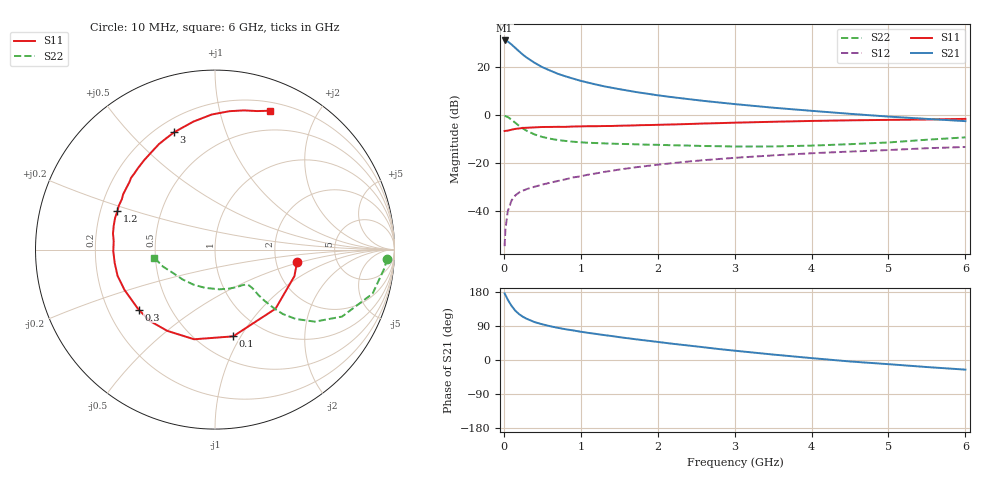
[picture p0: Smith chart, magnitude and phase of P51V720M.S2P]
! SIEMENS Small Signal Semiconductors
! BFP183
! Si NPN RF Bipolar Junction Transistor in SOT143
! VCE = 1.75 V  IC = 20 mA
! Common Emitter S-Parameters:  March  1996
# GHz  S  MA  R  50
!  f  S11  S21  S12  S22
! GHz  MAG  ANG  MAG  ANG  MAG  ANG  MAG  ANG
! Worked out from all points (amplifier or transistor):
!   36 points, 10 MHz to 6 GHz, reference 50 ohm
!   highest |S21| = 31.2 dB at 10 MHz (marker M1)
!   |S21| within 3 dB of that: start of sweep to 144.9 MHz
!   unconditionally stable (mu >= 1): 708.8 MHz to 5.69 GHz
!   at 250 MHz: K = 0.52, MSG = 28.4 dB, |S12| = -31.6 dB
!   at 1.4 GHz: K = 1.18, MAG = 14.8 dB, |S12| = -23.3 dB
!   at 6 GHz: K = 0.95, MSG = 5.4 dB, |S12| = -13.4 dB
!   S11 on the Smith chart (normalised r, x): 10 MHz: 2.62, -0.48; 100 MHz: 0.73, -0.93; 300 MHz: 0.33, -0.31; 1.2 GHz: 0.27, +0.18; 3 GHz: 0.27, +0.68; 6 GHz: 0.29, +1.43
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0.01  0.4625 -8.9  36.43 175.8  0.0018 85.4  0.9599 -3.0
0.02  0.4665 -18.5  36.34 171.9  0.0039 88.4  0.9494 -6.3
0.05  0.4714 -44.3  34.85 159.5  0.0095 78.8  0.9117 -15.6
0.1  0.4938 -78.2  29.99 142.8  0.0163 62.3  0.8002 -27.8
0.15  0.513 -103.1  25.35 130.0  0.0209 54.8  0.6862 -35.8
0.2  0.525 -120.4  21.41 120.7  0.024 51.7  0.5924 -40.7
0.25  0.5383 -132.3  18.21 113.8  0.0262 48.8  0.5213 -43.5
0.3  0.5414 -141.9  15.84 108.5  0.0283 48.3  0.4661 -44.8
0.4  0.552 -156.0  12.4 100.0  0.0316 48.3  0.3925 -46.0
0.5  0.5622 -165.0  10.06 94.2  0.035 47.5  0.3483 -46.3
0.6  0.5638 -172.5  8.555 89.2  0.0383 49.8  0.3202 -46.0
0.7  0.5668 -179.1  7.327 85.0  0.0416 50.6  0.3004 -45.9
0.8  0.5663 175.2  6.478 81.2  0.0451 51.7  0.2872 -46.1
1.1  0.5841 162.3  4.75 71.5  0.0567 53.1  0.263 -48.0
1.2  0.5839 158.5  4.349 68.8  0.0601 53.1  0.2593 -49.0
1.7  0.6073 141.7  3.067 55.1  0.0801 51.9  0.2445 -56.7
2.2  0.6358 128.3  2.356 42.7  0.0988 48.7  0.2329 -67.3
3  0.6923 109.2  1.697 24.6  0.1272 41.9  0.2193 -89.2
3.5  0.7232 99.6  1.425 14.4  0.1431 37.7  0.2203 -105.0
4.5  0.7755 84.0  1.061 -3.9  0.1719 28.5  0.2457 -137.5
5.5  0.8067 73.1  0.831 -18.6  0.202 20.5  0.3047 -161.9
6  0.832 68.4  0.746 -25.4  0.2148 15.8  0.3409 -172.3
